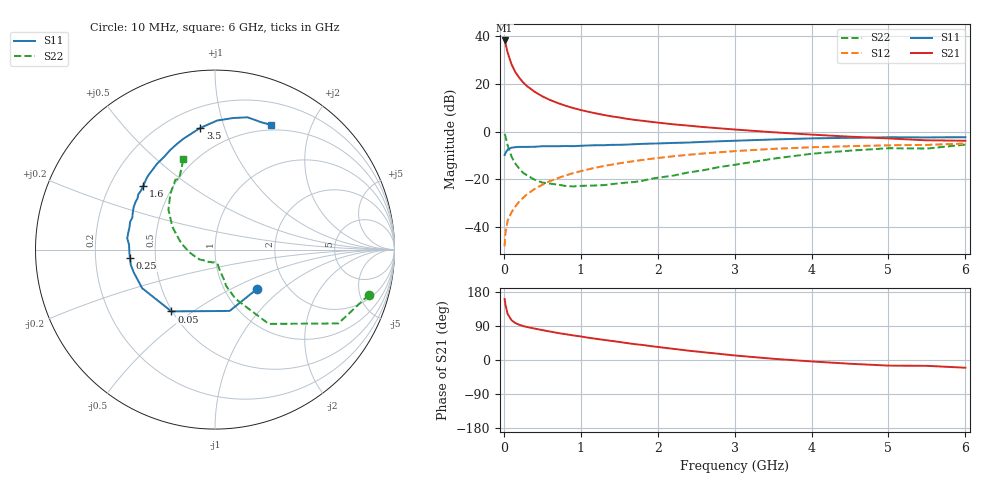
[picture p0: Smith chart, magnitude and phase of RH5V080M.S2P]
! SIEMENS Small Signal Semiconductors
! BFR106
! Si NPN RF Bipolar Junction Transistor in SOT23
! VCE = 5 V  IC = 80 mA
! Common Emitter S-Parameters:  August  1996
# GHz  S  MA  R  50
!  f  S11  S21  S12  S22
! GHz  MAG  ANG  MAG  ANG  MAG  ANG  MAG  ANG
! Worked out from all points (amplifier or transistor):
!   36 points, 10 MHz to 6 GHz, reference 50 ohm
!   highest |S21| = 38.3 dB at 10 MHz (marker M1)
!   |S21| within 3 dB of that: start of sweep to 33.9 MHz
!   unconditionally stable (mu >= 1): 206.8 MHz to 2.422 GHz
!   at 250 MHz: K = 1.04, MAG = 23.0 dB, |S12| = -27.9 dB
!   at 1.4 GHz: K = 1.06, MAG = 8.6 dB, |S12| = -13.9 dB
!   at 6 GHz: K = 0.99, MSG = 0.6 dB, |S12| = -5.0 dB
!   S11 on the Smith chart (normalised r, x): 10 MHz: 1.40, -0.69; 50 MHz: 0.49, -0.41; 250 MHz: 0.36, -0.04; 1.6 GHz: 0.34, +0.34; 3.5 GHz: 0.33, +0.83; 6 GHz: 0.44, +1.45
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0.01  0.3204 -43.8  82.45 161.2  0.0039 78.7  0.8934 -16.4
0.02  0.3513 -76.6  72.33 146.6  0.0074 69.7  0.8011 -30.9
0.05  0.4213 -125.2  45.55 121.1  0.0134 62.2  0.511 -54.1
0.1  0.4596 -152.2  25.95 105.1  0.0201 64.5  0.2976 -67.4
0.15  0.4702 -164.4  17.76 97.4  0.0267 67.3  0.2117 -73.0
0.2  0.4768 -169.7  13.55 93.1  0.0339 70.6  0.1668 -73.5
0.25  0.4764 -174.5  10.85 89.6  0.0405 72.1  0.1361 -75.7
0.3  0.4772 -177.5  9.082 87.2  0.0479 72.9  0.1209 -76.9
0.4  0.4798 176.7  6.879 82.9  0.0623 73.5  0.0974 -78.5
0.5  0.493 172.7  5.513 78.9  0.0763 73.3  0.0848 -79.5
0.6  0.4924 168.6  4.621 75.1  0.091 72.4  0.0807 -82.4
0.7  0.4925 165.1  3.991 71.4  0.105 71.9  0.0767 -86.9
0.9  0.4939 159.0  3.134 65.0  0.1339 69.2  0.0703 -93.4
1.1  0.5116 152.2  2.608 58.9  0.1613 66.7  0.0732 -104.4
1.3  0.5171 146.7  2.233 53.1  0.1887 63.7  0.0748 -114.5
1.6  0.5336 138.7  1.858 44.7  0.2279 59.4  0.0848 -131.1
2.2  0.5775 123.9  1.425 29.5  0.3026 50.3  0.1186 -161.7
2.8  0.6253 109.9  1.173 16.3  0.3677 41.0  0.1794 172.4
3.5  0.683 96.9  0.969 3.3  0.4338 30.5  0.2693 151.9
4.5  0.7399 82.2  0.782 -9.9  0.4935 15.9  0.3977 128.7
5.5  0.755 69.8  0.655 -15.4  0.5255 6.4  0.4402 117.1
6  0.7616 65.9  0.643 -20.4  0.5615 -0.8  0.5324 109.3
